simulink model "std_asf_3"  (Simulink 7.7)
settings: Solver=ode45  StartTime=0.0  StopTime=10.0  RelTol=1e-3

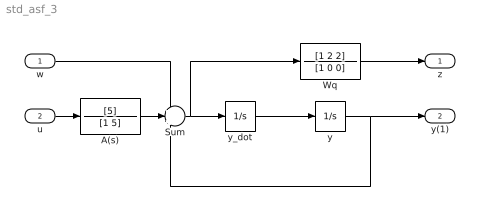
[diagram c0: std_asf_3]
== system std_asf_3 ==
  w : Inport
  u : Inport  Port=2
  A(s) : TransferFcn  Numerator=[5]  Denominator=[1 5]
  Sum : Sum  Inputs=+++
  Wq : TransferFcn  Numerator=[1 2 2]  Denominator=[1 0 0]
  y : Integrator
  y_dot : Integrator  InitialCondition=-1
  z : Outport
  y(1) : Outport  Port=2
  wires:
  Sum/1 -> y_dot/1, Wq/1
  y_dot/1 -> y/1
  y/1 -> Sum/3, y(1)/1
  Wq/1 -> z/1
  w/1 -> Sum/1
  u/1 -> A(s)/1
  A(s)/1 -> Sum/2
